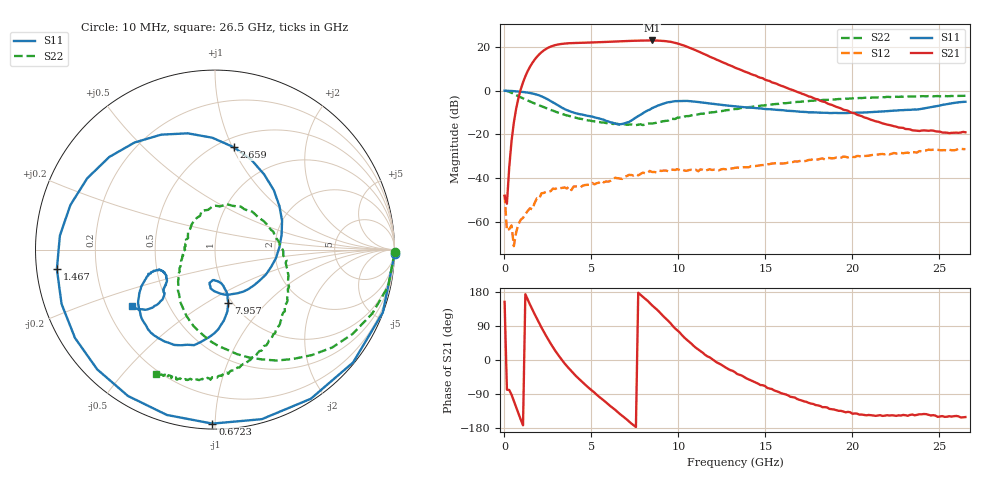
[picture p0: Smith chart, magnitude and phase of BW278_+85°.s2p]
!Agilent Technologies,N5242A,MY52422126,A.09.90.01
!Agilent N5242A: A.09.90.01
!Date: Wednesday, January 15, 2014 09:27:32
!Correction: S11(Full 2 Port with power(1,2))
!S21(Full 2 Port with power(1,2))
!S12(Full 2 Port with power(1,2))
!S22(Full 2 Port with power(1,2))
!S2P File: Measurements: S11, S21, S12, S22:
# Hz S  dB  R 50
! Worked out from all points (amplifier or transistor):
!   201 points, 10 MHz to 26.5 GHz, reference 50 ohm
!   highest |S21| = 23.1 dB at 8.487 GHz (marker M1)
!   |S21| within 3 dB of that: 2.606 GHz to 10.54 GHz (7.932 GHz wide, 121 % of centre)
!   unconditionally stable (mu >= 1): 141.6 MHz to end of sweep
!   at 4.381 GHz: K = 5.70, MAG = 22.6 dB, |S12| = -44.2 dB
!   at 13.26 GHz: K = 6.08, MAG = 12.2 dB, |S12| = -35.4 dB
!   at 26.5 GHz: K = 27.54, MAG = -13.5 dB, |S12| = -26.8 dB
!   S11 on the Smith chart (normalised r, x): 10 MHz: -4, -88; 672.2 MHz: 0.03, -0.98; 1.467 GHz: 0.06, -0.06; 2.659 GHz: 0.59, +1.01; 7.957 GHz: 0.96, -0.63; 26.5 GHz: 0.31, -0.28
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1e7  0.01 -1.3  -48.24 153.5  -47.59 -74.1  0.01 -0.9
6.7225e8  -0.27 -90.9  -8.30 -124.9  -65.02 46.1  -1.97 -47.5
1.46695e9  -1.03 -173.0  10.96 146.5  -53.92 -177.0  -4.99 -82.8
1.8643e9  -1.77 150.8  15.54 109.4  -49.36 149.4  -6.27 -97.0
2.1292e9  -2.54 126.9  17.66 85.8  -47.06 136.0  -7.09 -105.8
2.659e9  -4.73 79.7  20.26 43.3  -46.05 108.9  -8.79 -120.4
3.05635e9  -6.64 45.2  21.19 15.5  -44.45 100.0  -9.96 -129.2
3.4537e9  -8.39 12.7  21.64 -8.6  -44.38 80.7  -11.00 -136.5
4.5133e9  -11.00 -56.4  22.02 -59.5  -43.51 71.7  -13.06 -152.6
5.308e9  -12.46 -87.4  22.23 -91.8  -42.41 62.5  -14.21 -163.0
6.1027e9  -14.50 -99.5  22.51 -122.1  -41.29 59.8  -14.86 -171.5
7.1623e9  -14.32 -79.2  22.85 -162.2  -38.61 44.9  -15.52 169.9
7.957e9  -10.33 -75.9  23.02 166.6  -37.56 34.9  -15.74 156.8
8.4868e9  -7.99 -82.9  23.08 144.2  -37.27 27.5  -15.07 145.5
8.88415e9  -6.62 -90.5  22.99 127.8  -36.64 21.9  -14.36 132.9
9.67885e9  -4.94 -109.7  22.23 89.8  -36.23 14.2  -12.90 105.4
1.0606e10  -4.73 -130.1  19.87 49.0  -36.40 2.1  -11.61 68.2
1.16656e10  -5.66 -145.3  16.21 9.6  -36.34 -1.2  -10.24 33.3
1.3255e10  -7.17 -155.2  10.60 -32.3  -35.37 -11.1  -8.38 -1.8
1.77583e10  -9.88 -158.6  -3.35 -116.1  -31.28 -44.9  -4.60 -59.2
2.212915e10  -9.26 -144.0  -15.75 -146.5  -29.19 -87.0  -2.84 -92.1
2.65e10  -5.06 -145.8  -19.05 -150.6  -26.82 -135.2  -2.32 -115.4
